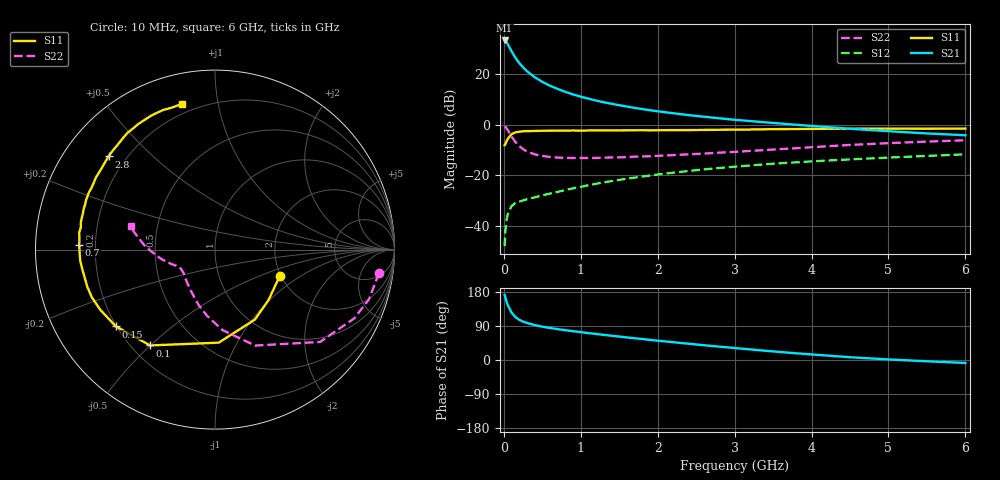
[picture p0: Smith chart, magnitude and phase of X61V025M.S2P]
! SIEMENS Small Signal Semiconductors
! BFP193W
! Si NPN RF Bipolar Junction Transistor in SOT343
! VCE = 1 V  IC = 25 mA
! Common Emitter S-Parameters:  April 1994
# GHz  S  MA  R  50
!  f  S11  S21  S12  S22
! GHz  MAG  ANG  MAG  ANG  MAG  ANG  MAG  ANG
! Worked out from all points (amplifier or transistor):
!   40 points, 10 MHz to 6 GHz, reference 50 ohm
!   highest |S21| = 33.3 dB at 10 MHz (marker M1)
!   |S21| within 3 dB of that: start of sweep to 77.66 MHz
!   unconditionally stable (mu >= 1): 729.9 MHz to 5.805 GHz
!   at 200 MHz: K = 0.44, MSG = 27.5 dB, |S12| = -30.6 dB
!   at 1.5 GHz: K = 1.17, MAG = 12.3 dB, |S12| = -21.9 dB
!   at 6 GHz: K = 0.99, MSG = 3.8 dB, |S12| = -11.8 dB
!   S11 on the Smith chart (normalised r, x): 10 MHz: 1.97, -0.69; 100 MHz: 0.27, -0.50; 150 MHz: 0.20, -0.33; 700 MHz: 0.14, +0.02; 2.8 GHz: 0.13, +0.37; 6 GHz: 0.15, +0.79
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0.01  0.3894 -22.3  46.27 171.6  0.0039 84.5  0.9229 -8.2
0.02  0.4098 -43.3  45.42 164.8  0.0078 73.9  0.9012 -17.9
0.03  0.4488 -60.3  43.77 157.8  0.0115 70.7  0.8652 -26.3
0.05  0.5189 -87.7  39.14 145.4  0.0168 61.0  0.7793 -41.3
0.1  0.6448 -124.1  28.37 125.1  0.0243 45.3  0.5796 -67.3
0.15  0.6985 -142.2  21.12 113.3  0.0279 39.5  0.4505 -84.6
0.2  0.7216 -152.2  16.54 106.3  0.0296 37.4  0.3735 -96.5
0.25  0.7359 -158.8  13.58 101.4  0.0315 36.9  0.3268 -105.5
0.3  0.7411 -163.7  11.4 97.8  0.0331 38.0  0.2926 -112.8
0.4  0.7454 -170.4  8.684 92.2  0.0361 40.5  0.2572 -123.5
0.5  0.7533 -175.2  7.012 88.0  0.0395 43.4  0.239 -131.1
0.6  0.7547 -178.8  5.86 84.5  0.043 45.6  0.228 -136.8
0.7  0.7577 177.9  5.074 81.5  0.0465 47.8  0.2216 -140.8
0.9  0.7627 172.9  3.95 76.0  0.0546 51.1  0.2177 -146.4
1.1  0.763 168.6  3.258 71.0  0.0629 53.4  0.2173 -150.2
1.6  0.7699 158.8  2.271 59.5  0.0847 55.3  0.2264 -155.1
2.2  0.7757 148.7  1.675 47.0  0.1113 54.1  0.2481 -160.4
2.8  0.7884 138.8  1.33 35.3  0.1378 50.9  0.2775 -165.3
3.2  0.7972 132.7  1.173 28.0  0.1545 48.4  0.3002 -169.5
4.5  0.8267 115.5  0.826 7.3  0.204 39.1  0.3945 176.5
5.5  0.8268 106.9  0.667 -3.4  0.2391 32.6  0.4592 168.0
6  0.8328 102.6  0.614 -7.8  0.2571 29.6  0.4877 164.6
